TYPE Warning :
STRUCT
	PRESSURE:BOOL;
	MFC1:BOOL;
	WALL_TEMP:BOOL;
	LID_TEMP:BOOL;
	STAGE_TEMP1:BOOL;
	STAGE_TEMP2:BOOL;
	STAGE_TEMP3:BOOL;
	STAGE_TEMP4:BOOL;
	OpenCloseSlitValveTimeout:BOOL;
	Gas1FlowPressureOutOfRange:BOOL;
	//PROCESS TOLERANCE
	TOLERANCE_PRESSURE:BOOL;
	TOLERANCE_MFC1:BOOL;
	TOLERANCE_WALL_TEMP:BOOL;
	TOLERANCE_LID_TEMP:BOOL;
	TOLERANCE_STAGE_TEMP1,
	TOLERANCE_STAGE_TEMP2,
	TOLERANCE_STAGE_TEMP3,
	TOLERANCE_STAGE_TEMP4: BOOL;	
END_STRUCT
END_TYPE
